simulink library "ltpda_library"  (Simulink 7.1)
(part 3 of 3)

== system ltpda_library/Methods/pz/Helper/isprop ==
  In1 : Inport  OutDataType=sfix(16)  OutScaling=2^0
  isprop : M-S-Function  Tag=isprop  FunctionName=ltpdasim
  Out1 : Outport  OutDataType=sfix(16)  OutScaling=2^0
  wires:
  In1/1 -> isprop/1
  isprop/1 -> Out1/1

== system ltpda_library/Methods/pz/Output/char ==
  In1 : Inport  OutDataType=sfix(16)  OutScaling=2^0
  Terminator : Terminator
  char : M-S-Function  Tag=char  FunctionName=ltpdasim
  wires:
  char/1 -> Terminator/1
  In1/1 -> char/1

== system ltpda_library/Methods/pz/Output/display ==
  In1 : Inport  OutDataType=sfix(16)  OutScaling=2^0
  Terminator : Terminator
  display : M-S-Function  Tag=display  FunctionName=ltpdasim
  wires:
  display/1 -> Terminator/1
  In1/1 -> display/1

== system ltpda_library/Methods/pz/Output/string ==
  In1 : Inport  OutDataType=sfix(16)  OutScaling=2^0
  Terminator : Terminator
  string : M-S-Function  Tag=string  FunctionName=ltpdasim
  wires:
  string/1 -> Terminator/1
  In1/1 -> string/1

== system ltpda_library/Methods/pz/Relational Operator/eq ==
  In1 : Inport  OutDataType=sfix(16)  OutScaling=2^0
  eq : M-S-Function  Tag=eq  FunctionName=ltpdasim
  Out1 : Outport  OutDataType=sfix(16)  OutScaling=2^0
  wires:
  In1/1 -> eq/1
  eq/1 -> Out1/1

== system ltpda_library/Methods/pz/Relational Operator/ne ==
  In1 : Inport  OutDataType=sfix(16)  OutScaling=2^0
  ne : M-S-Function  Tag=ne  FunctionName=ltpdasim
  Out1 : Outport  OutDataType=sfix(16)  OutScaling=2^0
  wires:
  In1/1 -> ne/1
  ne/1 -> Out1/1

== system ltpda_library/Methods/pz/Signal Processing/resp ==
  In1 : Inport  OutDataType=sfix(16)  OutScaling=2^0
  resp : M-S-Function  Tag=resp  FunctionName=ltpdasim
  Out1 : Outport  OutDataType=sfix(16)  OutScaling=2^0
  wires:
  In1/1 -> resp/1
  resp/1 -> Out1/1

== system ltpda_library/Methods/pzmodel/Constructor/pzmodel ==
  Ground : Ground
  pzmodel : M-S-Function  Tag=pzmodel  FunctionName=ltpdasim
  Out1 : Outport  OutDataType=sfix(16)  OutScaling=2^0
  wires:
  Ground/1 -> pzmodel/1
  pzmodel/1 -> Out1/1

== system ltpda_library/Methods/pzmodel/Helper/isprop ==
  In1 : Inport  OutDataType=sfix(16)  OutScaling=2^0
  isprop : M-S-Function  Tag=isprop  FunctionName=ltpdasim
  Out1 : Outport  OutDataType=sfix(16)  OutScaling=2^0
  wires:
  In1/1 -> isprop/1
  isprop/1 -> Out1/1

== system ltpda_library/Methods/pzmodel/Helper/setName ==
  In1 : Inport  OutDataType=sfix(16)  OutScaling=2^0
  setName : M-S-Function  Tag=setName  FunctionName=ltpdasim
  Out1 : Outport  OutDataType=sfix(16)  OutScaling=2^0
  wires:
  In1/1 -> setName/1
  setName/1 -> Out1/1

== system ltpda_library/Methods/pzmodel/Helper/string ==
  In1 : Inport  OutDataType=sfix(16)  OutScaling=2^0
  string : M-S-Function  Tag=string  FunctionName=ltpdasim
  Out1 : Outport  OutDataType=sfix(16)  OutScaling=2^0
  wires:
  In1/1 -> string/1
  string/1 -> Out1/1

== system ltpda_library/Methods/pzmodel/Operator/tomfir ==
  In1 : Inport  OutDataType=sfix(16)  OutScaling=2^0
  tomfir : M-S-Function  Tag=tomfir  FunctionName=ltpdasim
  Out1 : Outport  OutDataType=sfix(16)  OutScaling=2^0
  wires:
  In1/1 -> tomfir/1
  tomfir/1 -> Out1/1

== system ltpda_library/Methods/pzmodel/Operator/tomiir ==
  In1 : Inport  OutDataType=sfix(16)  OutScaling=2^0
  tomiir : M-S-Function  Tag=tomiir  FunctionName=ltpdasim
  Out1 : Outport  OutDataType=sfix(16)  OutScaling=2^0
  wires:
  In1/1 -> tomiir/1
  tomiir/1 -> Out1/1

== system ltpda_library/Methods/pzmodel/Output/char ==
  In1 : Inport  OutDataType=sfix(16)  OutScaling=2^0
  Terminator : Terminator
  char : M-S-Function  Tag=char  FunctionName=ltpdasim
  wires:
  char/1 -> Terminator/1
  In1/1 -> char/1

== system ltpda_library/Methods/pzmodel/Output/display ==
  In1 : Inport  OutDataType=sfix(16)  OutScaling=2^0
  Terminator : Terminator
  display : M-S-Function  Tag=display  FunctionName=ltpdasim
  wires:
  display/1 -> Terminator/1
  In1/1 -> display/1

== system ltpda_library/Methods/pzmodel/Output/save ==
  In1 : Inport  OutDataType=sfix(16)  OutScaling=2^0
  Terminator : Terminator
  save : M-S-Function  Tag=save  FunctionName=ltpdasim
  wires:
  save/1 -> Terminator/1
  In1/1 -> save/1

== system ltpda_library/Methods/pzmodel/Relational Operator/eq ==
  In1 : Inport  OutDataType=sfix(16)  OutScaling=2^0
  eq : M-S-Function  Tag=eq  FunctionName=ltpdasim
  Out1 : Outport  OutDataType=sfix(16)  OutScaling=2^0
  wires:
  In1/1 -> eq/1
  eq/1 -> Out1/1

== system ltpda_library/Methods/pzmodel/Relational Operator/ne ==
  In1 : Inport  OutDataType=sfix(16)  OutScaling=2^0
  ne : M-S-Function  Tag=ne  FunctionName=ltpdasim
  Out1 : Outport  OutDataType=sfix(16)  OutScaling=2^0
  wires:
  In1/1 -> ne/1
  ne/1 -> Out1/1

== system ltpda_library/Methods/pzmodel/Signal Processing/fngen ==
  In1 : Inport  OutDataType=sfix(16)  OutScaling=2^0
  fngen : M-S-Function  Tag=fngen  FunctionName=ltpdasim
  Out1 : Outport  OutDataType=sfix(16)  OutScaling=2^0
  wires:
  In1/1 -> fngen/1
  fngen/1 -> Out1/1

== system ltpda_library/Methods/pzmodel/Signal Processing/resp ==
  In1 : Inport  OutDataType=sfix(16)  OutScaling=2^0
  resp : M-S-Function  Tag=resp  FunctionName=ltpdasim
  Out1 : Outport  OutDataType=sfix(16)  OutScaling=2^0
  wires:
  In1/1 -> resp/1
  resp/1 -> Out1/1

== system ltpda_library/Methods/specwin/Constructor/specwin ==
  Ground : Ground
  specwin : M-S-Function  Tag=specwin  FunctionName=ltpdasim
  Out1 : Outport  OutDataType=sfix(16)  OutScaling=2^0
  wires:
  Ground/1 -> specwin/1
  specwin/1 -> Out1/1

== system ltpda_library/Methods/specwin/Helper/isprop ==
  In1 : Inport  OutDataType=sfix(16)  OutScaling=2^0
  isprop : M-S-Function  Tag=isprop  FunctionName=ltpdasim
  Out1 : Outport  OutDataType=sfix(16)  OutScaling=2^0
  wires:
  In1/1 -> isprop/1
  isprop/1 -> Out1/1

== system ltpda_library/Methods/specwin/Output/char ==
  In1 : Inport  OutDataType=sfix(16)  OutScaling=2^0
  Terminator : Terminator
  char : M-S-Function  Tag=char  FunctionName=ltpdasim
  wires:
  char/1 -> Terminator/1
  In1/1 -> char/1

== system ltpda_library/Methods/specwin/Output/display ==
  In1 : Inport  OutDataType=sfix(16)  OutScaling=2^0
  Terminator : Terminator
  display : M-S-Function  Tag=display  FunctionName=ltpdasim
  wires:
  display/1 -> Terminator/1
  In1/1 -> display/1

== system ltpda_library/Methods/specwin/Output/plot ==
  In1 : Inport  OutDataType=sfix(16)  OutScaling=2^0
  Terminator : Terminator
  plot : M-S-Function  Tag=plot  FunctionName=ltpdasim
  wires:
  plot/1 -> Terminator/1
  In1/1 -> plot/1

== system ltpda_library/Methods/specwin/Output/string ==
  In1 : Inport  OutDataType=sfix(16)  OutScaling=2^0
  Terminator : Terminator
  string : M-S-Function  Tag=string  FunctionName=ltpdasim
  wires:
  string/1 -> Terminator/1
  In1/1 -> string/1

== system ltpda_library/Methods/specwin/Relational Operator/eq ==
  In1 : Inport  OutDataType=sfix(16)  OutScaling=2^0
  eq : M-S-Function  Tag=eq  FunctionName=ltpdasim
  Out1 : Outport  OutDataType=sfix(16)  OutScaling=2^0
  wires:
  In1/1 -> eq/1
  eq/1 -> Out1/1

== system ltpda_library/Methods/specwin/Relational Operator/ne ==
  In1 : Inport  OutDataType=sfix(16)  OutScaling=2^0
  ne : M-S-Function  Tag=ne  FunctionName=ltpdasim
  Out1 : Outport  OutDataType=sfix(16)  OutScaling=2^0
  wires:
  In1/1 -> ne/1
  ne/1 -> Out1/1

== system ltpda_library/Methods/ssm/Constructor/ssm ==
  Ground : Ground
  ssm : M-S-Function  Tag=ssm  FunctionName=ltpdasim
  Out1 : Outport  OutDataType=sfix(16)  OutScaling=2^0
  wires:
  Ground/1 -> ssm/1
  ssm/1 -> Out1/1

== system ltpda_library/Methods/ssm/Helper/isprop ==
  In1 : Inport  OutDataType=sfix(16)  OutScaling=2^0
  isprop : M-S-Function  Tag=isprop  FunctionName=ltpdasim
  Out1 : Outport  OutDataType=sfix(16)  OutScaling=2^0
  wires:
  In1/1 -> isprop/1
  isprop/1 -> Out1/1

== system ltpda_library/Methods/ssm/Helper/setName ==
  In1 : Inport  OutDataType=sfix(16)  OutScaling=2^0
  setName : M-S-Function  Tag=setName  FunctionName=ltpdasim
  Out1 : Outport  OutDataType=sfix(16)  OutScaling=2^0
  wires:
  In1/1 -> setName/1
  setName/1 -> Out1/1

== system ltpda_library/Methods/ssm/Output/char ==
  In1 : Inport  OutDataType=sfix(16)  OutScaling=2^0
  Terminator : Terminator
  char : M-S-Function  Tag=char  FunctionName=ltpdasim
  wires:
  char/1 -> Terminator/1
  In1/1 -> char/1

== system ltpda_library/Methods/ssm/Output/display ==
  In1 : Inport  OutDataType=sfix(16)  OutScaling=2^0
  Terminator : Terminator
  display : M-S-Function  Tag=display  FunctionName=ltpdasim
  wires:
  display/1 -> Terminator/1
  In1/1 -> display/1

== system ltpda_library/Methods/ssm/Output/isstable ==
  In1 : Inport  OutDataType=sfix(16)  OutScaling=2^0
  Terminator : Terminator
  isstable : M-S-Function  Tag=isstable  FunctionName=ltpdasim
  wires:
  isstable/1 -> Terminator/1
  In1/1 -> isstable/1

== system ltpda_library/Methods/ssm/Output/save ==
  In1 : Inport  OutDataType=sfix(16)  OutScaling=2^0
  Terminator : Terminator
  save : M-S-Function  Tag=save  FunctionName=ltpdasim
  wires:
  save/1 -> Terminator/1
  In1/1 -> save/1

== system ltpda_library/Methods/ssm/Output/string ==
  In1 : Inport  OutDataType=sfix(16)  OutScaling=2^0
  Terminator : Terminator
  string : M-S-Function  Tag=string  FunctionName=ltpdasim
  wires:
  string/1 -> Terminator/1
  In1/1 -> string/1

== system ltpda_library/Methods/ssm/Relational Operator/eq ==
  In1 : Inport  OutDataType=sfix(16)  OutScaling=2^0
  eq : M-S-Function  Tag=eq  FunctionName=ltpdasim
  Out1 : Outport  OutDataType=sfix(16)  OutScaling=2^0
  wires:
  In1/1 -> eq/1
  eq/1 -> Out1/1

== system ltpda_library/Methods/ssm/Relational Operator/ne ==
  In1 : Inport  OutDataType=sfix(16)  OutScaling=2^0
  ne : M-S-Function  Tag=ne  FunctionName=ltpdasim
  Out1 : Outport  OutDataType=sfix(16)  OutScaling=2^0
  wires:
  In1/1 -> ne/1
  ne/1 -> Out1/1

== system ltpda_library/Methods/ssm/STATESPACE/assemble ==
  In1 : Inport  OutDataType=sfix(16)  OutScaling=2^0
  assemble : M-S-Function  Tag=assemble  FunctionName=ltpdasim
  Out1 : Outport  OutDataType=sfix(16)  OutScaling=2^0
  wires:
  In1/1 -> assemble/1
  assemble/1 -> Out1/1

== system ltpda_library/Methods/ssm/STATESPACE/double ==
  In1 : Inport  OutDataType=sfix(16)  OutScaling=2^0
  double : M-S-Function  Tag=double  FunctionName=ltpdasim
  Out1 : Outport  OutDataType=sfix(16)  OutScaling=2^0
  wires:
  In1/1 -> double/1
  double/1 -> Out1/1

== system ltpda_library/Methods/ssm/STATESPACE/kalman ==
  In1 : Inport  OutDataType=sfix(16)  OutScaling=2^0
  kalman : M-S-Function  Tag=kalman  FunctionName=ltpdasim
  Out1 : Outport  OutDataType=sfix(16)  OutScaling=2^0
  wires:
  In1/1 -> kalman/1
  kalman/1 -> Out1/1

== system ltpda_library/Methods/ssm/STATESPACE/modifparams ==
  In1 : Inport  OutDataType=sfix(16)  OutScaling=2^0
  modifparams : M-S-Function  Tag=modifparams  FunctionName=ltpdasim
  Out1 : Outport  OutDataType=sfix(16)  OutScaling=2^0
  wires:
  In1/1 -> modifparams/1
  modifparams/1 -> Out1/1

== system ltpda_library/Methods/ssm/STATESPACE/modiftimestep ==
  In1 : Inport  OutDataType=sfix(16)  OutScaling=2^0
  modiftimestep : M-S-Function  Tag=modiftimestep  FunctionName=ltpdasim
  Out1 : Outport  OutDataType=sfix(16)  OutScaling=2^0
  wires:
  In1/1 -> modiftimestep/1
  modiftimestep/1 -> Out1/1

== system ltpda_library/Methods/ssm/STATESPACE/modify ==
  In1 : Inport  OutDataType=sfix(16)  OutScaling=2^0
  modify : M-S-Function  Tag=modify  FunctionName=ltpdasim
  Out1 : Outport  OutDataType=sfix(16)  OutScaling=2^0
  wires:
  In1/1 -> modify/1
  modify/1 -> Out1/1

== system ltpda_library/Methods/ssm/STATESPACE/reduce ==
  In1 : Inport  OutDataType=sfix(16)  OutScaling=2^0
  reduce : M-S-Function  Tag=reduce  FunctionName=ltpdasim
  Out1 : Outport  OutDataType=sfix(16)  OutScaling=2^0
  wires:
  In1/1 -> reduce/1
  reduce/1 -> Out1/1

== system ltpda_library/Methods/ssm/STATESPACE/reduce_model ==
  In1 : Inport  OutDataType=sfix(16)  OutScaling=2^0
  reduce_model : M-S-Function  Tag=reduce_model  FunctionName=ltpdasim
  Out1 : Outport  OutDataType=sfix(16)  OutScaling=2^0
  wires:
  In1/1 -> reduce_model/1
  reduce_model/1 -> Out1/1

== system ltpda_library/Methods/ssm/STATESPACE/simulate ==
  In1 : Inport  OutDataType=sfix(16)  OutScaling=2^0
  simulate : M-S-Function  Tag=simulate  FunctionName=ltpdasim
  Out1 : Outport  OutDataType=sfix(16)  OutScaling=2^0
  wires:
  In1/1 -> simulate/1
  simulate/1 -> Out1/1

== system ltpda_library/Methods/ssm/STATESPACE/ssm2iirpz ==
  In1 : Inport  OutDataType=sfix(16)  OutScaling=2^0
  ssm2iirpz : M-S-Function  Tag=ssm2iirpz  FunctionName=ltpdasim
  Out1 : Outport  OutDataType=sfix(16)  OutScaling=2^0
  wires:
  In1/1 -> ssm2iirpz/1
  ssm2iirpz/1 -> Out1/1

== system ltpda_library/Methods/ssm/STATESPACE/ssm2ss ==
  In1 : Inport  OutDataType=sfix(16)  OutScaling=2^0
  ssm2ss : M-S-Function  Tag=ssm2ss  FunctionName=ltpdasim
  Out1 : Outport  OutDataType=sfix(16)  OutScaling=2^0
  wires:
  In1/1 -> ssm2ss/1
  ssm2ss/1 -> Out1/1

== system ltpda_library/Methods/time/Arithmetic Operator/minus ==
  In1 : Inport  OutDataType=sfix(16)  OutScaling=2^0
  minus : M-S-Function  Tag=minus  FunctionName=ltpdasim
  Out1 : Outport  OutDataType=sfix(16)  OutScaling=2^0
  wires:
  In1/1 -> minus/1
  minus/1 -> Out1/1

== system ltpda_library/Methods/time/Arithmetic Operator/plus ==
  In1 : Inport  OutDataType=sfix(16)  OutScaling=2^0
  plus : M-S-Function  Tag=plus  FunctionName=ltpdasim
  Out1 : Outport  OutDataType=sfix(16)  OutScaling=2^0
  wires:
  In1/1 -> plus/1
  plus/1 -> Out1/1

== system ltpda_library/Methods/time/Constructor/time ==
  Ground : Ground
  time : M-S-Function  Tag=time  FunctionName=ltpdasim
  Out1 : Outport  OutDataType=sfix(16)  OutScaling=2^0
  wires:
  Ground/1 -> time/1
  time/1 -> Out1/1

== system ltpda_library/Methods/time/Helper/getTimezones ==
  In1 : Inport  OutDataType=sfix(16)  OutScaling=2^0
  getTimezones : M-S-Function  Tag=getTimezones  FunctionName=ltpdasim
  Out1 : Outport  OutDataType=sfix(16)  OutScaling=2^0
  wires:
  In1/1 -> getTimezones/1
  getTimezones/1 -> Out1/1

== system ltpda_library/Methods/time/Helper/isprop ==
  In1 : Inport  OutDataType=sfix(16)  OutScaling=2^0
  isprop : M-S-Function  Tag=isprop  FunctionName=ltpdasim
  Out1 : Outport  OutDataType=sfix(16)  OutScaling=2^0
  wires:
  In1/1 -> isprop/1
  isprop/1 -> Out1/1

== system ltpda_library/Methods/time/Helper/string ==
  In1 : Inport  OutDataType=sfix(16)  OutScaling=2^0
  string : M-S-Function  Tag=string  FunctionName=ltpdasim
  Out1 : Outport  OutDataType=sfix(16)  OutScaling=2^0
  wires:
  In1/1 -> string/1
  string/1 -> Out1/1

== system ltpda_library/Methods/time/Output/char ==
  In1 : Inport  OutDataType=sfix(16)  OutScaling=2^0
  Terminator : Terminator
  char : M-S-Function  Tag=char  FunctionName=ltpdasim
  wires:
  char/1 -> Terminator/1
  In1/1 -> char/1

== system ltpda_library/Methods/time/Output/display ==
  In1 : Inport  OutDataType=sfix(16)  OutScaling=2^0
  Terminator : Terminator
  display : M-S-Function  Tag=display  FunctionName=ltpdasim
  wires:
  display/1 -> Terminator/1
  In1/1 -> display/1

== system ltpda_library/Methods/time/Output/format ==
  In1 : Inport  OutDataType=sfix(16)  OutScaling=2^0
  Terminator : Terminator
  format : M-S-Function  Tag=format  FunctionName=ltpdasim
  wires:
  format/1 -> Terminator/1
  In1/1 -> format/1

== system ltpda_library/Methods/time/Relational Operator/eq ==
  In1 : Inport  OutDataType=sfix(16)  OutScaling=2^0
  eq : M-S-Function  Tag=eq  FunctionName=ltpdasim
  Out1 : Outport  OutDataType=sfix(16)  OutScaling=2^0
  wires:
  In1/1 -> eq/1
  eq/1 -> Out1/1

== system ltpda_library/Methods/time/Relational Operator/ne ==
  In1 : Inport  OutDataType=sfix(16)  OutScaling=2^0
  ne : M-S-Function  Tag=ne  FunctionName=ltpdasim
  Out1 : Outport  OutDataType=sfix(16)  OutScaling=2^0
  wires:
  In1/1 -> ne/1
  ne/1 -> Out1/1

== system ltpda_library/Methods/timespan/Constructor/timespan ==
  Ground : Ground
  timespan : M-S-Function  Tag=timespan  FunctionName=ltpdasim
  Out1 : Outport  OutDataType=sfix(16)  OutScaling=2^0
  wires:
  Ground/1 -> timespan/1
  timespan/1 -> Out1/1

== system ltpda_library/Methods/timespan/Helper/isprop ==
  In1 : Inport  OutDataType=sfix(16)  OutScaling=2^0
  isprop : M-S-Function  Tag=isprop  FunctionName=ltpdasim
  Out1 : Outport  OutDataType=sfix(16)  OutScaling=2^0
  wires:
  In1/1 -> isprop/1
  isprop/1 -> Out1/1

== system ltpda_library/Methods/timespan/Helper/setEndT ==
  In1 : Inport  OutDataType=sfix(16)  OutScaling=2^0
  setEndT : M-S-Function  Tag=setEndT  FunctionName=ltpdasim
  Out1 : Outport  OutDataType=sfix(16)  OutScaling=2^0
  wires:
  In1/1 -> setEndT/1
  setEndT/1 -> Out1/1

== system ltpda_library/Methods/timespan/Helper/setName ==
  In1 : Inport  OutDataType=sfix(16)  OutScaling=2^0
  setName : M-S-Function  Tag=setName  FunctionName=ltpdasim
  Out1 : Outport  OutDataType=sfix(16)  OutScaling=2^0
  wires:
  In1/1 -> setName/1
  setName/1 -> Out1/1

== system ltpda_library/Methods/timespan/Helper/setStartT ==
  In1 : Inport  OutDataType=sfix(16)  OutScaling=2^0
  setStartT : M-S-Function  Tag=setStartT  FunctionName=ltpdasim
  Out1 : Outport  OutDataType=sfix(16)  OutScaling=2^0
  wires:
  In1/1 -> setStartT/1
  setStartT/1 -> Out1/1

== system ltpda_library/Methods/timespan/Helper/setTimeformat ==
  In1 : Inport  OutDataType=sfix(16)  OutScaling=2^0
  setTimeformat : M-S-Function  Tag=setTimeformat  FunctionName=ltpdasim
  Out1 : Outport  OutDataType=sfix(16)  OutScaling=2^0
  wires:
  In1/1 -> setTimeformat/1
  setTimeformat/1 -> Out1/1

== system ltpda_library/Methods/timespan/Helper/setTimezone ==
  In1 : Inport  OutDataType=sfix(16)  OutScaling=2^0
  setTimezone : M-S-Function  Tag=setTimezone  FunctionName=ltpdasim
  Out1 : Outport  OutDataType=sfix(16)  OutScaling=2^0
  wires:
  In1/1 -> setTimezone/1
  setTimezone/1 -> Out1/1

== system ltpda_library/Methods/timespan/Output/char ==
  In1 : Inport  OutDataType=sfix(16)  OutScaling=2^0
  Terminator : Terminator
  char : M-S-Function  Tag=char  FunctionName=ltpdasim
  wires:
  char/1 -> Terminator/1
  In1/1 -> char/1

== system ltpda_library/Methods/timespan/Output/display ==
  In1 : Inport  OutDataType=sfix(16)  OutScaling=2^0
  Terminator : Terminator
  display : M-S-Function  Tag=display  FunctionName=ltpdasim
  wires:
  display/1 -> Terminator/1
  In1/1 -> display/1

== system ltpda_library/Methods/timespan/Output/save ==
  In1 : Inport  OutDataType=sfix(16)  OutScaling=2^0
  Terminator : Terminator
  save : M-S-Function  Tag=save  FunctionName=ltpdasim
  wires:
  save/1 -> Terminator/1
  In1/1 -> save/1

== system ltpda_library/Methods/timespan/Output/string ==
  In1 : Inport  OutDataType=sfix(16)  OutScaling=2^0
  Terminator : Terminator
  string : M-S-Function  Tag=string  FunctionName=ltpdasim
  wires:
  string/1 -> Terminator/1
  In1/1 -> string/1

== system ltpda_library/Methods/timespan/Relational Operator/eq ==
  In1 : Inport  OutDataType=sfix(16)  OutScaling=2^0
  eq : M-S-Function  Tag=eq  FunctionName=ltpdasim
  Out1 : Outport  OutDataType=sfix(16)  OutScaling=2^0
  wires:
  In1/1 -> eq/1
  eq/1 -> Out1/1

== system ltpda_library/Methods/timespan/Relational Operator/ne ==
  In1 : Inport  OutDataType=sfix(16)  OutScaling=2^0
  ne : M-S-Function  Tag=ne  FunctionName=ltpdasim
  Out1 : Outport  OutDataType=sfix(16)  OutScaling=2^0
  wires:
  In1/1 -> ne/1
  ne/1 -> Out1/1

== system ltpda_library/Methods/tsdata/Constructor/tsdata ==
  Ground : Ground
  tsdata : M-S-Function  Tag=tsdata  FunctionName=ltpdasim
  Out1 : Outport  OutDataType=sfix(16)  OutScaling=2^0
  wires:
  Ground/1 -> tsdata/1
  tsdata/1 -> Out1/1

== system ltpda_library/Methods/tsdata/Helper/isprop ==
  In1 : Inport  OutDataType=sfix(16)  OutScaling=2^0
  isprop : M-S-Function  Tag=isprop  FunctionName=ltpdasim
  Out1 : Outport  OutDataType=sfix(16)  OutScaling=2^0
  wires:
  In1/1 -> isprop/1
  isprop/1 -> Out1/1

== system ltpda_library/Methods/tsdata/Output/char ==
  In1 : Inport  OutDataType=sfix(16)  OutScaling=2^0
  Terminator : Terminator
  char : M-S-Function  Tag=char  FunctionName=ltpdasim
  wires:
  char/1 -> Terminator/1
  In1/1 -> char/1

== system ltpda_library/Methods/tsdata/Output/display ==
  In1 : Inport  OutDataType=sfix(16)  OutScaling=2^0
  Terminator : Terminator
  display : M-S-Function  Tag=display  FunctionName=ltpdasim
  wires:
  display/1 -> Terminator/1
  In1/1 -> display/1

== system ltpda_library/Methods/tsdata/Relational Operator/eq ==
  In1 : Inport  OutDataType=sfix(16)  OutScaling=2^0
  eq : M-S-Function  Tag=eq  FunctionName=ltpdasim
  Out1 : Outport  OutDataType=sfix(16)  OutScaling=2^0
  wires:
  In1/1 -> eq/1
  eq/1 -> Out1/1

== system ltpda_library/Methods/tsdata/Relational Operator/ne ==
  In1 : Inport  OutDataType=sfix(16)  OutScaling=2^0
  ne : M-S-Function  Tag=ne  FunctionName=ltpdasim
  Out1 : Outport  OutDataType=sfix(16)  OutScaling=2^0
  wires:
  In1/1 -> ne/1
  ne/1 -> Out1/1

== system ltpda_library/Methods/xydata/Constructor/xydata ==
  Ground : Ground
  xydata : M-S-Function  Tag=xydata  FunctionName=ltpdasim
  Out1 : Outport  OutDataType=sfix(16)  OutScaling=2^0
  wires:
  Ground/1 -> xydata/1
  xydata/1 -> Out1/1

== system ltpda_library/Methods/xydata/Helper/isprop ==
  In1 : Inport  OutDataType=sfix(16)  OutScaling=2^0
  isprop : M-S-Function  Tag=isprop  FunctionName=ltpdasim
  Out1 : Outport  OutDataType=sfix(16)  OutScaling=2^0
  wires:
  In1/1 -> isprop/1
  isprop/1 -> Out1/1

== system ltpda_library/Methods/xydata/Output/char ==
  In1 : Inport  OutDataType=sfix(16)  OutScaling=2^0
  Terminator : Terminator
  char : M-S-Function  Tag=char  FunctionName=ltpdasim
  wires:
  char/1 -> Terminator/1
  In1/1 -> char/1

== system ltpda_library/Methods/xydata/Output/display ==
  In1 : Inport  OutDataType=sfix(16)  OutScaling=2^0
  Terminator : Terminator
  display : M-S-Function  Tag=display  FunctionName=ltpdasim
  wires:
  display/1 -> Terminator/1
  In1/1 -> display/1

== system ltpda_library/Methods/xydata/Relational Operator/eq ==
  In1 : Inport  OutDataType=sfix(16)  OutScaling=2^0
  eq : M-S-Function  Tag=eq  FunctionName=ltpdasim
  Out1 : Outport  OutDataType=sfix(16)  OutScaling=2^0
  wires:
  In1/1 -> eq/1
  eq/1 -> Out1/1

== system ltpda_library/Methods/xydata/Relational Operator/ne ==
  In1 : Inport  OutDataType=sfix(16)  OutScaling=2^0
  ne : M-S-Function  Tag=ne  FunctionName=ltpdasim
  Out1 : Outport  OutDataType=sfix(16)  OutScaling=2^0
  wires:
  In1/1 -> ne/1
  ne/1 -> Out1/1

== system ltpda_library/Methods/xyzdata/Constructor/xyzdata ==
  Ground : Ground
  xyzdata : M-S-Function  Tag=xyzdata  FunctionName=ltpdasim
  Out1 : Outport  OutDataType=sfix(16)  OutScaling=2^0
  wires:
  Ground/1 -> xyzdata/1
  xyzdata/1 -> Out1/1

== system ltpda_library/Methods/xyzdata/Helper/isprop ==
  In1 : Inport  OutDataType=sfix(16)  OutScaling=2^0
  isprop : M-S-Function  Tag=isprop  FunctionName=ltpdasim
  Out1 : Outport  OutDataType=sfix(16)  OutScaling=2^0
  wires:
  In1/1 -> isprop/1
  isprop/1 -> Out1/1

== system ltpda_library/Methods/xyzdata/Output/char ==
  In1 : Inport  OutDataType=sfix(16)  OutScaling=2^0
  Terminator : Terminator
  char : M-S-Function  Tag=char  FunctionName=ltpdasim
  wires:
  char/1 -> Terminator/1
  In1/1 -> char/1

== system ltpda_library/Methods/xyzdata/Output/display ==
  In1 : Inport  OutDataType=sfix(16)  OutScaling=2^0
  Terminator : Terminator
  display : M-S-Function  Tag=display  FunctionName=ltpdasim
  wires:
  display/1 -> Terminator/1
  In1/1 -> display/1

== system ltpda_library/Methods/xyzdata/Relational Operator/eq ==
  In1 : Inport  OutDataType=sfix(16)  OutScaling=2^0
  eq : M-S-Function  Tag=eq  FunctionName=ltpdasim
  Out1 : Outport  OutDataType=sfix(16)  OutScaling=2^0
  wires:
  In1/1 -> eq/1
  eq/1 -> Out1/1

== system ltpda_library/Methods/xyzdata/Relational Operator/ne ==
  In1 : Inport  OutDataType=sfix(16)  OutScaling=2^0
  ne : M-S-Function  Tag=ne  FunctionName=ltpdasim
  Out1 : Outport  OutDataType=sfix(16)  OutScaling=2^0
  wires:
  In1/1 -> ne/1
  ne/1 -> Out1/1
